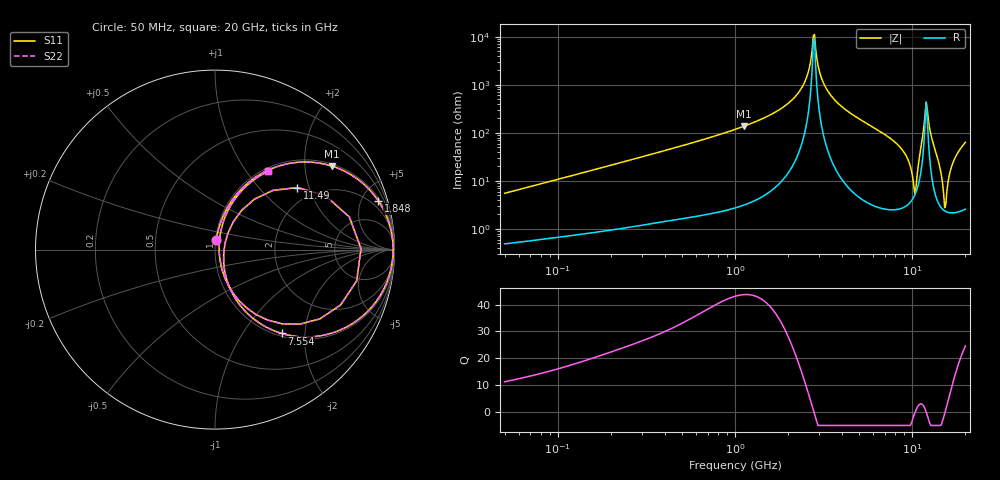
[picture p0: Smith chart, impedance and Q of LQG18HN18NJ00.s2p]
!Murata Part Number: LQG18HN18NJ00
!These Parameters are Measured in Series Mode Connection
!  o--[Z]--o
!Port1  Port2
!  o-------o
!Freq. Start=50[MHz] Stop=20[GHz], 401[Steps]
# Hz S RI R 50
!Freq.(Hz) S11(Real) S11(Imag) S21(Real) S21(Imag) S12(Real) S12(Imag) S22(Real) S22(Imag)
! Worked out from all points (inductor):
!   401 points, 50 MHz to 20 GHz, reference 50 ohm
!   read as one part in series: L = 17.3 nH near 51.52 MHz
!   highest Q = 43.7 at 1.127 GHz (marker M1), where L = 19.5 nH
!   self-resonance near 2.769 GHz
!   S11 on the Smith chart (normalised r, x): 50 MHz: 1.01, +0.11; 1.848 GHz: 1.20, +6.64; 7.554 GHz: 1.05, -1.52; 11.49 GHz: 1.63, +1.68; 20 GHz: 1.05, +1.27
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5e7  0.00782 0.0543  0.9922 -0.0543  0.9922 -0.0543  0.00782 0.0543
1.364002e8  0.0281 0.1407  0.9719 -0.1407  0.9719 -0.1407  0.0281 0.1407
3.721004e8  0.144 0.3343  0.856 -0.3343  0.856 -0.3343  0.144 0.3343
1e9  0.5795 0.4822  0.4205 -0.4822  0.4205 -0.4822  0.5795 0.4822
1.127304e9  0.6525 0.4649  0.3475 -0.4649  0.3475 -0.4649  0.6525 0.4649
1.848039e9  0.9099 0.2714  0.0901 -0.2714  0.0901 -0.2714  0.9099 0.2714
2.419936e9  0.982 0.1007  0.018 -0.1007  0.018 -0.1007  0.982 0.1007
2.728004e9  0.9923 0.0166  0.00773 -0.0166  0.00773 -0.0166  0.9923 0.0166
2.853386e9  0.9923 -0.0157  0.00768 0.0157  0.00768 0.0157  0.9923 -0.0157
3.168813e9  0.9839 -0.0917  0.0161 0.0917  0.0161 0.0917  0.9839 -0.0917
3.680849e9  0.95 -0.1996  0.05 0.1996  0.05 0.1996  0.95 -0.1996
7.442007e9  0.39 -0.4722  0.61 0.4722  0.61 0.4722  0.39 -0.4722
7.554318e9  0.3714 -0.467  0.6286 0.467  0.6286 0.467  0.3714 -0.467
9.178299e9  0.1299 -0.297  0.8701 0.297  0.8701 0.297  0.1299 -0.297
1.034674e10  0.0484 -0.02  0.9516 0.02  0.9516 0.02  0.0484 -0.02
1.149051e10  0.4594 0.3458  0.5406 -0.3458  0.5406 -0.3458  0.4594 0.3458
1.201863e10  0.8137 0.00539  0.1863 -0.00539  0.1863 -0.00539  0.8137 0.00539
1.276073e10  0.4721 -0.4154  0.5279 0.4154  0.5279 0.4154  0.4721 -0.4154
1.417136e10  0.0775 -0.2052  0.9225 0.2052  0.9225 0.2052  0.0775 -0.2052
1.527346e10  0.0234 -0.0137  0.9766 0.0137  0.9766 0.0137  0.0234 -0.0137
1.721783e10  0.0833 0.2386  0.9167 -0.2386  0.9167 -0.2386  0.0833 0.2386
2e10  0.2957 0.4365  0.7043 -0.4365  0.7043 -0.4365  0.2957 0.4365
